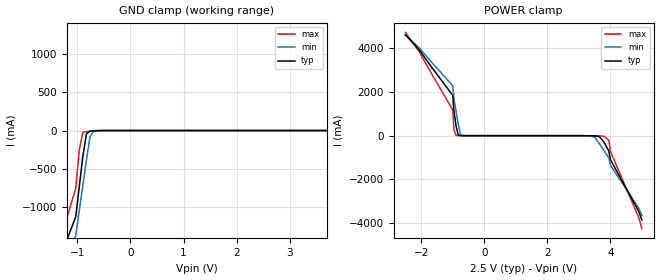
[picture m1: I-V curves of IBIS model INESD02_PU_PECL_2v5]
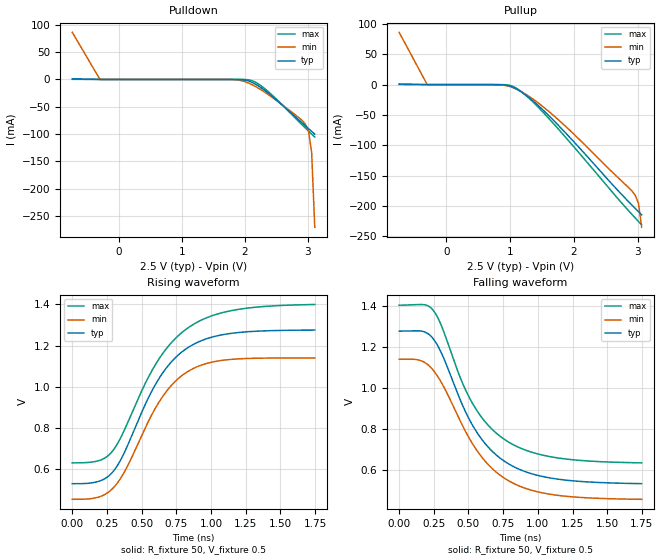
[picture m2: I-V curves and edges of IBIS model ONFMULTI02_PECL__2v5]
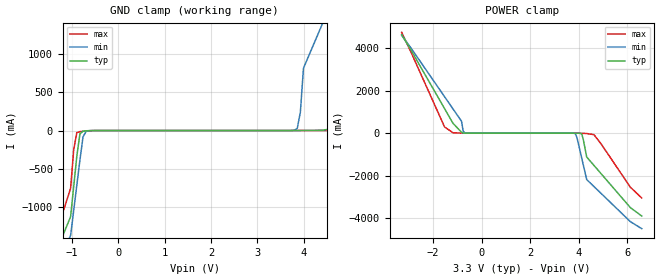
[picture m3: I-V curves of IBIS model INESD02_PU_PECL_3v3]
|   This file is an IBIS representation of the   |
|   Integrated Device Technology , Inc.   |
|   83PR226I-01   |
|   PROGRAMMABLE FEMTOCLOCK LVPECL OSCILLATOR REPLACEMENT   |
[IBIS Ver]   4.1
[File name]   83pr226i_01.ibs
[File Rev]   1.0
[Date]   27 May 2010
[Source]   Originated at Integrated Device Technology, Inc.
[Disclaimer]
IDT hereby grants the user of this IBIS model a non-exclusive,
nontransferable license to use this IBIS model under the following terms.
Before using this IBIS model, the user should read this license.
If the user does not accept these terms,  the IBIS model should be
returned to IDT within 30 days.
   The user is granted this license only to use the IBIS model and
is not granted rights to sell, load, rent, lease or license the IBIS
model in whole or in part, or in modified form to anyone other than
user. User may modify the IBIS model to suit its specific
applications but rights to derivative works and such modifications
shall belong to IDT.
   This IBIS model is provided on an "AS IS" basis and IDT makes
absolutely no warranty with respect to the information contained
herein. IDT DISCLAIMS AND CUSTOMER WAIVES ALL WARRANTIES, EXPRESS
OR IMPLIED, INCLUDING WARRANTIES OF MERCHANTABILITY OR FITNESS FOR
A PARTICULAR PURPOSE. The entire risk as to quality and performance
is with the Customer. ACCORDINGLY, IN NO EVENT SHALL THE COMPANY BE
LIABLE FOR ANY DAMAGES, WHETHER IN CONTRACT OR TORT,INCLUDING ANY
LOST PROFITS OR OTHER INCIDENTAL, CONSEQUENTIAL, EXEMPLARY, OR
PUNITIVE DAMAGES ARISING OUT OF THE USE OR APPLICATION OF THE IBIS
model provided in this package. Further, IDT reserves the right to
make changes without notice to any product herein to improve
reliability, function, or design. IDT does not convey any license
under patent rights or any other intellectual property rights,
including those of third parties.
   IDT is not obligated to provide maintenance or support
for the licensed IBIS model.
[Copyright]   Copyright 2010 by Integrated Device Technology , Inc.
[Component]   83PR226KI-01
[Manufacturer] Integrated Device Technology, Inc.
[Package]
|VFQFN 10 Lead
|   typ   min   max
R_pkg   97.2824m   65.7555m   122.0734m
L_pkg   0.3877n   0.3190n   0.4764n
C_pkg   0.0767p   0.0569p   0.0979p
[Pin]   signal_name   model_name   R_pin   L_pin   C_pin
1   M1   INESD02_PU_PECL   122.0735m   0.3732n   0.0979p
2   M0   INESD02_PU_PECL   71.0181m   0.3190n   0.0784p
3   VEE   GND   107.0351m   0.4274n   0.0964p
4   XTAL_IN   NC   105.1539m   0.3523n   0.0621p
5   XTAL_OUT   NC   109.9892m   0.4744n   0.0628p
6   Q   ONFMULTI02_PECL_   101.2420m   0.3244n   0.0909p
7   nQ   ONFMULTI02_PECL_   65.7555m   0.3335n   0.0733p
8   VCC   POWER   93.3010m   0.4719n   0.0869p
9   N1   INESD02_PU_PECL   117.5016m   0.3250n   0.0610p
10  NO   INESD02_PU_PECL   79.7533m   0.4764n   0.0569p
[Diff Pin]   inv_pin   vdiff   tdelay_typ   tdelay_min   tdelay_max
6   7   NA   0   0   0
5   4   0.15   NA   NA   NA
[Model Selector] INESD02_PU_PECL
INESD02_PU_PECL_2v5  Buffer selection for 2v5
INESD02_PU_PECL_3v3  Buffer selection for 3v3
[Model Selector] ONFMULTI02_PECL_
ONFMULTI02_PECL__2v5  Buffer selection for 2v5
ONFMULTI02_PECL__3v3  Buffer selection for 3v3
| Models and submodels in the file (4): INESD02_PU_PECL_2v5 (Input), ONFMULTI02_PECL__2v5 (Output_ECL), INESD02_PU_PECL_3v3 (Input), ONFMULTI02_PECL__3v3 (Output_ECL)
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[Model] INESD02_PU_PECL_2v5
Model_type   Input
Polarity   Non-Inverting
Vinl = .8V
Vinh =  2V
|   typ   min   max
C_comp   2pF   1.5pF   2.5pF
|   typ   min   max
[Voltage range]  2.5V   2.375V   2.625V
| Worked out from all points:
|   GND clamp passes 1 mA (typ) near -0.59 V on its own axis
|   POWER clamp passes 1 mA (typ) near -0.70 V on its own axis
[GND_clamp]
|Voltage   I(typ)   I(min)   I(max)
-2.5V     -3.894A    -3.674A    -4.294A
-1.25V    -1.521A    -1.7A      -1.261A
-1.031V   -1.125A    -1.372A    -755.3mA
-896.9mV  -335.4mA   -714.7mA   -27.06mA
-695.9mV  -3.401mA   -10.7mA    -6.467mA
3.995V    711.6uA    10.32mA    481.3uA
4.062V    4.029mA    88.04mA    1.401mA
4.129V    40.44mA    547.3mA    3.341mA
4.196V    445.8mA    1.124A     14.79mA
4.263V    1.139A     1.7A       275.9mA
4.5V      1.832A     2.277A     1.163A
5V        3.219A     3.431A     2.937A
[POWER_clamp]
|Voltage   I(typ)   I(min)   I(max)
-2.5V     4.617A     4.594A     4.726A
-1V       1.842A     2.286A     1.176A
-963.9mV  1.149A     1.709A     289.6mA
-896.9mV  456.4mA    1.132A     15.33mA
-829.9mV  42.02mA    556.1mA    3.389mA
-762.9mV  4.159mA    91.01mA    1.421mA
-695.9mV  727.9uA    10.67mA    490.4uA
3.35V     -3.204mA   -9.193mA   -6.2mA
3.8V      -305mA     -689.5mA   -24.7mA
3.95V     -699.9mA   -1.018A    -211mA
4V        -1.095A    -1.346A    -716.4mA
5V        -3.863A    -3.649A    -4.255A
[Model] ONFMULTI02_PECL__2v5
Model_type   Output_ECL
Polarity   Non-Inverting
|   typ   min   max
C_comp   2pF   1.5pF   2.5pF
Vmeas = 0.86V
Rref = 50
Cref = 0
Vref = 0.5V
|   typ   min   max
[Voltage range]   2.5V   2.375V   2.625V
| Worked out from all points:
|   rising waveform, R_fixture 50, V_fixture 0.5: 20-80 % time 348ps typ, 329ps min, 389ps max; typ from 0.531 V to 1.27 V
|   falling waveform, R_fixture 50, V_fixture 0.5: 20-80 % time 353ps typ, 369ps min, 350ps max; typ from 1.28 V to 0.534 V
[Pulldown]
|Voltage   I (typ)   I (min)   I (max)
|Note, modeling breaks down at 250mA and above.  This is well beyond the functional   |
|operating range of the device.  Should this scenario occur, catastrophic failure and   |
|possible damage to the device and/or board is of higher concern than the I-V curve   |
|behavior.  The IBIS checker will flag currents in excess of 10A with warnings.  Lines   |
|with currents in excess of 0.35 A have been commented out.  The points still remain|
|available to the user if the user desires to use them.   |
|-2.06000e+00   3.85620e+00   3.24774e+00   4.55908e+00
|-1.62000e+00   2.44790e+00   2.19088e+00   2.76152e+00
|-1.18000e+00   1.04259e+00   1.13638e+00   9.67359e-01
-740mV    1.109mA    86.21mA    135.6uA
-300mV    30.91nA    4.721uA    118pA
1.781V    -4.494uA   -148.8uA   -45.78nA
1.929V    -264.5uA   -1.816mA   -21.25uA
2.077V    -3.491mA   -7.461mA   -1.083mA
2.176V    -8.945mA   -13.19mA   -5.369mA
2.323V    -20.47mA   -23.75mA   -17.4mA
2.866V    -74.82mA   -70.54mA   -77.83mA
2.964V    -84.94mA   -81.99mA   -88.99mA
3.014V    -90.01mA   -94.74mA   -94.52mA
3.063V    -95.1mA    -133.7mA   -100mA
3.112V    -100.2mA   -270.4mA   -105.5mA
| 3.16172e+00   -1.05409e-01   -4.55628e-01   -1.10884e-01
| 3.21103e+00   -1.10832e-01   -6.40833e-01   -1.16317e-01
| 3.26034e+00   -1.17703e-01   -8.26048e-01   -1.21768e-01
| 3.30966e+00   -1.34353e-01   -1.01127e+00   -1.27247e-01
| 3.35897e+00   -2.17604e-01   -1.19655e+00   -1.32752e-01
| 3.40828e+00   -4.58138e-01   -1.38187e+00   -1.38291e-01
| 3.45759e+00   -7.04356e-01   -1.56721e+00   -1.44086e-01
| 3.50690e+00   -9.50678e-01   -1.75254e+00   -1.52835e-01
| 3.55621e+00   -1.19700e+00   -1.93787e+00   -1.96032e-01
| 3.60552e+00   -1.44331e+00   -2.12321e+00   -4.54298e-01
| 3.65483e+00   -1.68962e+00   -2.30854e+00   -7.68118e-01
| 3.70414e+00   -1.93592e+00   -2.49387e+00   -1.08192e+00
| 3.75345e+00   -2.18221e+00   -2.67920e+00   -1.39572e+00
| 3.80276e+00   -2.42850e+00   -2.86453e+00   -1.70950e+00
| 3.85207e+00   -2.67477e+00   -3.04985e+00   -2.02326e+00
| 3.90138e+00   -2.92105e+00   -3.23517e+00   -2.33702e+00
| 3.95069e+00   -3.16731e+00   -3.42049e+00   -2.65076e+00
| 4.00000e+00   -3.41357e+00   -3.60581e+00   -2.96450e+00
| 4.01000e+00   -3.46351e+00   -3.64339e+00   -3.02812e+00
| 4.20800e+00   -4.45228e+00   -4.38749e+00   -4.28781e+00
| 4.40600e+00   -5.44105e+00   -5.13161e+00   -5.54751e+00
| 4.60400e+00   -6.42992e+00   -5.87578e+00   -6.80742e+00
| 4.80200e+00   -7.41907e+00   -6.62011e+00   -8.06779e+00
| 5.00000e+00   -8.40870e+00   -7.36470e+00   -9.32899e+00
[Pullup]
|Voltage   I (typ)   I (min)   I (max)
|Note, modeling breaks down at 250mA and above.  This is well beyond the functional   |
|operating range of the device.  Should this scenario occur, catastrophic failure and   |
|possible damage to the device and/or board is of higher concern than the I-V curve   |
|behavior.  The IBIS checker will flag currents in excess of 10A with warnings.  Lines   |
|with currents in excess of 0.35 A have been commented out.  The points still remain|
|available to the user if the user desires to use them.   |
|-2.06000e+00   3.85620e+00   3.24774e+00   4.55908e+00
|-1.62000e+00   2.44790e+00   2.19088e+00   2.76152e+00
|-1.18000e+00   1.04259e+00   1.13638e+00   9.67359e-01
-740mV    1.109mA    86.21mA    135.6uA
-300mV    30.91nA    4.721uA    118pA
844.1mV   -108.6uA   -382uA     -19.85uA
992.1mV   -2.135mA   -3.112mA   -1.111mA
1.091V    -6.507mA   -7.078mA   -5.414mA
1.337V    -24.9mA    -22.28mA   -26.36mA
1.732V    -64.33mA   -55.56mA   -70.23mA
2.028V    -97.36mA   -84.43mA   -105.9mA
2.915V    -199mA     -175.8mA   -214.4mA
2.964V    -204.3mA   -182.7mA   -220mA
3.014V    -209.5mA   -195.7mA   -225.6mA
3.063V    -214.7mA   -234.9mA   -231.1mA
| 3.11241e+00   -2.19988e-01   -3.71984e-01   -2.36520e-01
| 3.16172e+00   -2.25287e-01   -5.57419e-01   -2.41951e-01
| 3.21103e+00   -2.30805e-01   -7.42852e-01   -2.47374e-01
| 3.26034e+00   -2.37761e-01   -9.28277e-01   -2.52809e-01
| 3.30966e+00   -2.54484e-01   -1.11369e+00   -2.58266e-01
| 3.35897e+00   -3.37801e-01   -1.29916e+00   -2.63746e-01
| 3.40828e+00   -5.78392e-01   -1.48468e+00   -2.69257e-01
| 3.45759e+00   -8.24663e-01   -1.67018e+00   -2.75023e-01
| 3.50690e+00   -1.07104e+00   -1.85568e+00   -2.83743e-01
| 3.55621e+00   -1.31741e+00   -2.04118e+00   -3.26909e-01
| 3.60552e+00   -1.56378e+00   -2.22666e+00   -5.85147e-01
| 3.65483e+00   -1.81013e+00   -2.41214e+00   -8.98943e-01
| 3.70414e+00   -2.05648e+00   -2.59762e+00   -1.21273e+00
| 3.75345e+00   -2.30281e+00   -2.78309e+00   -1.52650e+00
| 3.80276e+00   -2.54914e+00   -2.96855e+00   -1.84026e+00
| 3.85207e+00   -2.79546e+00   -3.15401e+00   -2.15400e+00
| 3.90138e+00   -3.04178e+00   -3.33947e+00   -2.46774e+00
| 3.95069e+00   -3.28809e+00   -3.52492e+00   -2.78146e+00
| 4.00000e+00   -3.53439e+00   -3.71037e+00   -3.09518e+00
| 4.01000e+00   -3.58434e+00   -3.74798e+00   -3.15879e+00
| 4.20800e+00   -4.57329e+00   -4.49261e+00   -4.41839e+00
| 4.40600e+00   -5.56220e+00   -5.23726e+00   -5.67791e+00
| 4.60400e+00   -6.55113e+00   -5.98196e+00   -6.93745e+00
| 4.80200e+00   -7.54015e+00   -6.72678e+00   -8.19711e+00
| 5.00000e+00   -8.52936e+00   -7.47177e+00   -9.45702e+00
[Ramp]
|   typ   min   max
dV/dt_r   0.446/0.347n   0.41/0.329n   0.46/0.388n
dV/dt_f   0.446/0.353n   0.409/0.369n   0.462/0.35n
R_load =   50.0000
[Rising Waveform]
R_fixture = 50
V_fixture = 0.5   | VCC_typ - 2V
V_fixture_max = 0.625   | VCC_max - 2V
V_fixture_min = 0.375   | VCC_min - 2V
C_fixture = 0.0p
| Time   typ   min   max
0s        530.9mV    455.3mV    632mV
190.9ps   542.6mV    466.4mV    642.7mV
292.5ps   588.5mV    508.7mV    691mV
385.4ps   696mV      599.6mV    805.3mV
518.5ps   903.8mV    790.7mV    1.006V
614.9ps   1.029V     914.8mV    1.125V
718.2ps   1.124V     1.01V      1.217V
837.3ps   1.192V     1.076V     1.287V
1.163ns   1.261V     1.134V     1.371V
1.748ns   1.275V     1.14V      1.399V
[Falling Waveform]
R_fixture = 50
V_fixture = 0.5   | VCC_typ - 2V
V_fixture_max = 0.625   | VCC_max - 2V
V_fixture_min = 0.375   | VCC_min - 2V
C_fixture = 0.0p
| Time   typ   min   max
0s        1.276V     1.139V     1.402V
152.4ps   1.277V     1.133V     1.405V
247ps     1.237V     1.085V     1.376V
301.3ps   1.174V     1.03V      1.308V
437.9ps   945.3mV    842.5mV    1.054V
522ps     826.4mV    735.6mV    932.4mV
635.9ps   716.2mV    631.2mV    822.5mV
770.8ps   637.7mV    555.3mV    743.9mV
1.116ns   558.6mV    479.6mV    662mV
1.748ns   534mV      457.8mV    635.1mV
[Model] INESD02_PU_PECL_3v3
Model_type  Input
Polarity   Non-Inverting
Vinl = 0.8V
Vinh = 2.0V
|   typ   min   max
C_comp   2pF   1.5pF   2.5pF
|   typ   min   max
[Voltage range]  3.3V   3.135V   3.465V
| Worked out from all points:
|   GND clamp passes 1 mA (typ) near -0.59 V on its own axis
|   POWER clamp passes 1 mA (typ) near -0.70 V on its own axis
[GND_clamp]
|Voltage   I(typ)   I(min)   I(max)
-3.3V     -3.894A    -3.674A    -4.294A
-1.3V     -1.521A    -1.7A      -1.261A
-1.031V   -1.125A    -1.372A    -755.3mA
-896.9mV  -335.4mA   -714.7mA   -27.07mA
-695.9mV  -3.401mA   -10.69mA   -6.477mA
3.794V    17.99uA    3.319mA    6.081uA
3.928V    181.1uA    239mA      10.12uA
3.995V    711.6uA    813.7mA    20.78uA
4.8V      40.44mA    1.967A     268.6uA
5.6V      1.139A     3.12A      2.243mA
6.3V      2.525A     4.275A     64.01mA
6.6V      3.219A     4.852A     752.7mA
[POWER_clamp]
|Voltage   I(typ)   I(min)   I(max)
-3.3V     4.617A     4.594A     4.726A
-1.53V    1.149A     1.709A     289.6mA
-1.18V    456.4mA    1.132A     15.33mA
-829.9mV  42.02mA    556.1mA    3.39mA
-762.9mV  4.159mA    91mA       1.422mA
-695.9mV  727.9uA    10.66mA    491.6uA
3.861V    -620.9uA   -26.2mA    -103.4uA
4.129V    -41.91mA   -1.19A     -4.968mA
4.33V     -1.119A    -2.176A    -17.93mA
4.63V     -1.515A    -2.505A    -71.45mA
6.13V     -3.492A    -4.151A    -2.536A
6.6V      -3.888A    -4.48A     -3.041A
